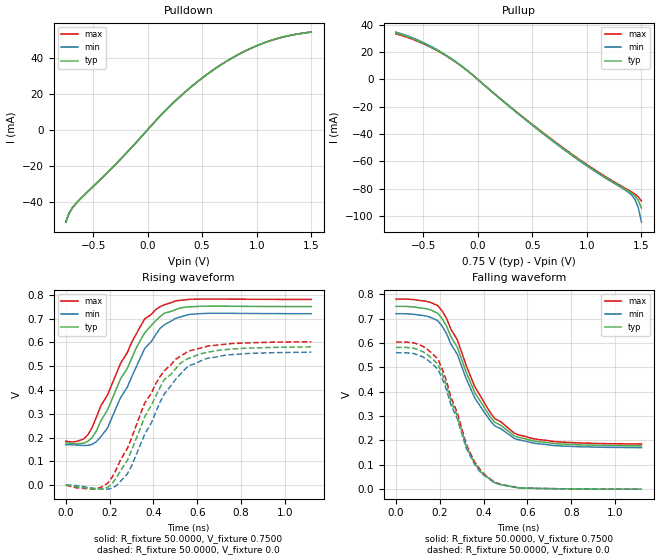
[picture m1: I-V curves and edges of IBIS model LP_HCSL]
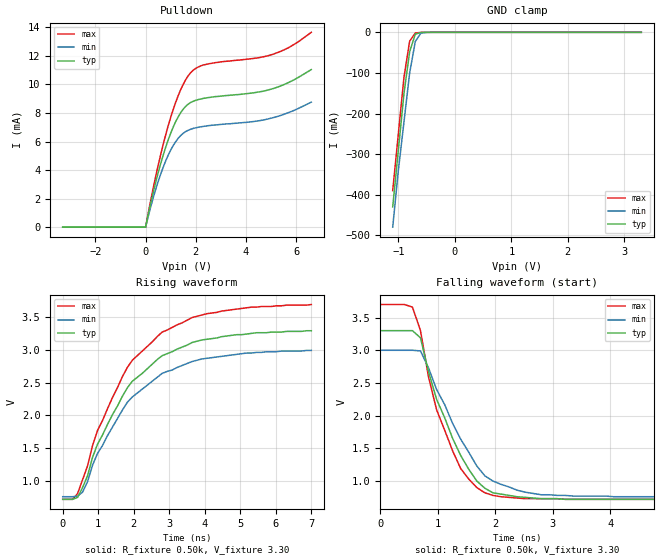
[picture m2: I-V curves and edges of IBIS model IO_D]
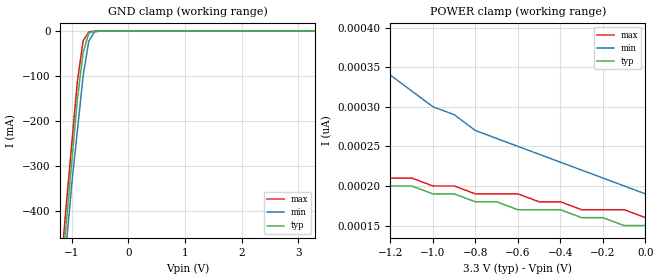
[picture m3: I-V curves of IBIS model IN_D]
| Integrated Devices Technolgy, Inc
[IBIS Ver]   4.1
[File name]   9zxl1530b.ibs
[File Rev]   1.3
|Rev history   1.3   Replace LP_HCSL model
[Date]   June 10, 2015
|[File Rev]   1.0
|Rev history   1.0   original revision
|[Date]   April 4, 2013
[Disclaimer] Integrated Device Technology, Inc. ("IDT") hereby grants the
   user of this ibis model a non-exclusive, nontransferable
   license to use this ibis model under the following terms. the
   user is granted this license only to use the ibis model and is
   not granted rights to sell, copy (except as needed to run the
   ibis model), rent, lease or sub-license the ibis model in
   whole or in part, or in modified form to anyone. the user may
   modify the ibis model to suit its specific applications, but
   rights to derivative works and such modifications shall belong
   to idt. this ibis model is provided on an as is" basis and idt
   makes absolutely no warranty with respect to the information
   contained herein. idt disclaims and customer waives all
   warranties, express and implied, including warranties of
   merchantability and fitness for a particular purpose. the
   entire risk as to quality and performance is with the user
   accordingly, in no event shall idt be liable for any direct or
   indirect damages, whether in contract or tort, including any
   lost profits or other incidental, consequential, exemplary, or
   punitive damages arising out of the use or application of the
   ibis model. further, idt reserves the right to make changes
   without notice to any product herein to improve reliability,
   function, or design. idt does not convey any license under
   patent rights or any other intellectual property rights,
   including those of third parties. idt is not obligated to
   provide maintenance or support for the licensed ibis model.
[Copyright]   Copyright 2012, Integrated Devices Technolgy, Inc. all rights
   reserved
[Notes]
   This file was modified on 6/10/2015 13:07 by the Mentor Graphics
   IBISVTC program, to remove initial non-switching delay(s) from one
   or more models V-t tables. Modified models:
   LP_HCSL,
   IO_D
   Original V-t tables have been left in the affected models, but commented out.
|   COMPONENT: 9ZXL1530B
[Component]   9ZXL1530B
[Manufacturer]   Integrated Device Technology, Inc.
[Package]
| variable   typ   min   max
R_pkg   81.10m   62.20m   100.00m
L_pkg   6.70nH   4.90nH   8.50nH
C_pkg   0.53pF   0.21pF   0.85pF
[Pin]   signal_name   model_name   R_pin   L_pin   C_pin
1   VDDA   POWER
2   GNDA   GND
3   100M_133M#   IN
4   HIBW_BYPM_LOBW#   IN
5   CKPWRGD_PD#   IN
6   GND   GND
7   VDDR   POWER
8   DIF_IN   DIFF_IN
9   DIF_IN#   DIFF_IN
10   SMB_A0_tri   IN
11   SMBDAT   IO_D
12   SMBCLK   IN_D
13   SMB_A1_tri   IN
14   FBOUT_NC#   LP_HCSL
15   FBOUT_NC   LP_HCSL
16   GND   GND
17   DIF_0   LP_HCSL
18   DIF_0#   LP_HCSL
19   VDDIO   POWER
20   GND   GND
21   DIF_1   LP_HCSL
22   DIF_1#   LP_HCSL
23   DIF_2   LP_HCSL
24   DIF_2#   LP_HCSL
25   GND   GND
26   VDD   POWER
27   DIF_3   LP_HCSL
28   DIF_3#   LP_HCSL
29   DIF_4   LP_HCSL
30   DIF_4#   LP_HCSL
31   VDDIO   POWER
32   GND   GND
33   DIF_5   LP_HCSL
34   DIF_5#   LP_HCSL
35   GND   GND
36   VDDIO   POWER
37   DIF_6   LP_HCSL
38   DIF_6#   LP_HCSL
39   DIF_7   LP_HCSL
40   DIF_7#   LP_HCSL
41   VDD   POWER
42   GND   GND
43   DIF_8   LP_HCSL
44   DIF_8#   LP_HCSL
45   DIF_9   LP_HCSL
46   DIF_9#   LP_HCSL
47   GND   GND
48   VDDIO   POWER
49   DIF_10   LP_HCSL
50   DIF_10#   LP_HCSL
51   VDDIO   POWER
52   GND   GND
53   DIF_11   LP_HCSL
54   DIF_11#   LP_HCSL
55   DIF_12   LP_HCSL
56   DIF_12#   LP_HCSL
57   GND   GND
58   VDD   POWER
59   DIF_13   LP_HCSL
60   DIF_13#   LP_HCSL
61   DIF_14   LP_HCSL
62   DIF_14#   LP_HCSL
63   VDDIO   POWER
64   GND   GND
[Diff Pin]   inv_pin   vdiff   tdelay_typ
8   9   NA   NA
15   14   NA   NA
17   18   NA   NA
21   22   NA   NA
23   24   NA   NA
27   28   NA   NA
29   30   NA   NA
33   34   NA   NA
37   38   NA   NA
39   40   NA   NA
43   44   NA   NA
45   46   NA   NA
49   50   NA   NA
53   54   NA   NA
55   56   NA   NA
59   60   NA   NA
61   62   NA   NA
| Models and submodels in the file (5): LP_HCSL (Output), IO_D (I/O_open_drain), IN_D (Input), IN (Input), DIFF_IN (Input)
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|   Model LP_HCSL
[Model]   LP_HCSL
Model_type Output
Polarity   Non-Inverting
Vmeas =  0.4000V
Cref =   2.0000pF
Rref =   0.0
Vref =   0.4000V
C_comp   1.1000pF   1.0000pF   1.2000pF
[Temperature Range]   25.0000   75.0000   0.0000
[Voltage Range]   0.7500V   0.7200V   0.7800V
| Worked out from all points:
|   slope of the pulldown table from 0 to 0.112 V, typ, clamps not added: 15.1 ohm
|   slope of the pullup table from 0 to 0.112 V, typ, clamps not added: 14.4 ohm
|   rising waveform, R_fixture 50.0000, V_fixture 0.7500: 20-80 % time 183ps typ, 186ps min, 189ps max; typ from 0.177 V to 0.75 V
|   rising waveform, R_fixture 50.0000, V_fixture 0.0: 20-80 % time 192ps typ, 189ps min, 192ps max; typ from 0 V to 0.581 V
|   falling waveform, R_fixture 50.0000, V_fixture 0.7500: 20-80 % time 188ps typ, 187ps min, 190ps max; typ from 0.75 V to 0.178 V
|   falling waveform, R_fixture 50.0000, V_fixture 0.0: 20-80 % time 139ps typ, 139ps min, 139ps max; typ from 0.582 V to 0 V
[Pulldown]
|Voltage   I(typ)   I(min)   I(max)
-750mV    -51.3mA    -51.29mA   -51.32mA
-720mV    -46.33mA   -46.32mA   -46.34mA
-690mV    -43.41mA   -43.4mA    -43.42mA
-630mV    -39.24mA   -39.23mA   -39.24mA
-240mV    -15.84mA   -15.84mA   -15.84mA
180mV     11.62mA    11.62mA    11.62mA
330mV     20.18mA    20.18mA    20.18mA
480mV     27.74mA    27.74mA    27.74mA
720mV     37.83mA    37.83mA    37.83mA
990mV     46.31mA    46.31mA    46.31mA
1.23V     51.24mA    51.24mA    51.24mA
1.5V      54.14mA    54.14mA    54.14mA
[Pullup]
|Voltage   I(typ)   I(min)   I(max)
-750mV    34.02mA    34.68mA    33.35mA
-480mV    25.87mA    26.28mA    25.45mA
-240mV    14.89mA    15.08mA    14.69mA
-90mV     6.064mA    6.135mA    5.992mA
360mV     -24.34mA   -24.59mA   -24.09mA
750mV     -48.65mA   -49.09mA   -48.19mA
1.08V     -67.16mA   -67.68mA   -66.63mA
1.38V     -81.8mA    -82.7mA    -81.06mA
1.41V     -83.41mA   -84.74mA   -82.5mA
1.44V     -85.42mA   -87.87mA   -84.07mA
1.47V     -88.51mA   -93.63mA   -86.04mA
1.5V      -94.23mA   -104.6mA   -89.1mA
[Ramp]
| variable   typ   min   max
dV/dt_r  0.3484/0.1898n   0.3352/0.1864n   0.3614/0.1921n
dV/dt_f  0.3432/0.1852n   0.3297/0.1833n   0.3567/0.1870n
R_load = 50.0000
[Rising Waveform]
R_fixture= 50.0000
V_fixture= 0.7500
V_fixture_min= 0.7200
V_fixture_max= 0.7800
|time   V(typ)   V(min)   V(max)
|0.0S   0.1772V   0.1698V   0.1847V
|22.22pS   0.1772V   0.1698V   0.1847V
|44.44pS   0.1772V   0.1698V   0.1847V
|66.67pS   0.1772V   0.1698V   0.1847V
|88.89pS   0.1772V   0.1698V   0.1847V
|0.11nS   0.1772V   0.1698V   0.1847V
|0.13nS   0.1772V   0.1698V   0.1847V
|0.16nS   0.1772V   0.1698V   0.1847V
|0.18nS   0.1772V   0.1698V   0.1847V
|0.20nS   0.1772V   0.1698V   0.1847V
|0.22nS   0.1772V   0.1698V   0.1847V
|0.24nS   0.1772V   0.1698V   0.1847V
|0.27nS   0.1772V   0.1698V   0.1847V
|0.29nS   0.1772V   0.1698V   0.1847V
|0.31nS   0.1772V   0.1698V   0.1847V
|0.33nS   0.1772V   0.1698V   0.1847V
|0.36nS   0.1772V   0.1698V   0.1847V
|0.38nS   0.1772V   0.1698V   0.1847V
|0.40nS   0.1772V   0.1698V   0.1847V
|0.42nS   0.1772V   0.1698V   0.1847V
|0.44nS   0.1772V   0.1698V   0.1847V
|0.47nS   0.1772V   0.1698V   0.1847V
|0.49nS   0.1772V   0.1698V   0.1847V
|0.51nS   0.1772V   0.1698V   0.1847V
|0.53nS   0.1772V   0.1698V   0.1847V
|0.56nS   0.1772V   0.1698V   0.1847V
|0.58nS   0.1772V   0.1698V   0.1847V
|0.60nS   0.1772V   0.1698V   0.1847V
|0.62nS   0.1772V   0.1698V   0.1847V
|0.64nS   0.1772V   0.1698V   0.1847V
|0.67nS   0.1772V   0.1698V   0.1847V
|0.69nS   0.1772V   0.1698V   0.1847V
|0.71nS   0.1772V   0.1698V   0.1847V
|0.73nS   0.1772V   0.1698V   0.1847V
|0.76nS   0.1772V   0.1698V   0.1847V
|0.78nS   0.1772V   0.1698V   0.1847V
|0.80nS   0.1772V   0.1698V   0.1847V
|0.82nS   0.1772V   0.1698V   0.1847V
|0.84nS   0.1772V   0.1698V   0.1847V
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0s        177.2mV    169.8mV    184.7mV
50.33ps   173.6mV    167.9mV    184.1mV
100.3ps   183.7mV    166.7mV    210.9mV
160.3ps   270.8mV    203.9mV    333.6mV
190.3ps   315.9mV    239.9mV    378.7mV
250.3ps   447.1mV    368.1mV    512.4mV
360.3ps   640.1mV    574.6mV    698.3mV
430.3ps   708.2mV    659mV      749.8mV
560.3ps   748.9mV    717mV      780.4mV
1.12ns    750.3mV    720.3mV    780.2mV
[Rising Waveform]
R_fixture= 50.0000
V_fixture= 0.0
V_fixture_min= 0.0
V_fixture_max= 0.0
|time   V(typ)   V(min)   V(max)
|0.0S   0.0V   0.0V   0.0V
|22.22pS   0.0V   0.0V   0.0V
|44.44pS   0.0V   0.0V   0.0V
|66.67pS   0.0V   0.0V   0.0V
|88.89pS   0.0V   0.0V   0.0V
|0.11nS   0.0V   0.0V   0.0V
|0.13nS   0.0V   0.0V   0.0V
|0.16nS   0.0V   0.0V   0.0V
|0.18nS   0.0V   0.0V   0.0V
|0.20nS   0.0V   0.0V   0.0V
|0.22nS   0.0V   0.0V   0.0V
|0.24nS   0.0V   0.0V   0.0V
|0.27nS   0.0V   0.0V   0.0V
|0.29nS   0.0V   0.0V   0.0V
|0.31nS   0.0V   0.0V   0.0V
|0.33nS   0.0V   0.0V   0.0V
|0.36nS   0.0V   0.0V   0.0V
|0.38nS   0.0V   0.0V   0.0V
|0.40nS   0.0V   0.0V   0.0V
|0.42nS   0.0V   0.0V   0.0V
|0.44nS   0.0V   0.0V   0.0V
|0.47nS   0.0V   0.0V   0.0V
|0.49nS   0.0V   0.0V   0.0V
|0.51nS   0.0V   0.0V   0.0V
|0.53nS   0.0V   0.0V   0.0V
|0.56nS   0.0V   0.0V   0.0V
|0.58nS   0.0V   0.0V   0.0V
|0.60nS   0.0V   0.0V   0.0V
|0.62nS   0.0V   0.0V   0.0V
|0.64nS   0.0V   0.0V   0.0V
|0.67nS   0.0V   0.0V   0.0V
|0.69nS   0.0V   0.0V   0.0V
|0.71nS   0.0V   0.0V   0.0V
|0.73nS   0.0V   0.0V   0.0V
|0.76nS   0.0V   0.0V   0.0V
|0.78nS   0.0V   0.0V   0.0V
|0.80nS   0.0V   0.0V   0.0V
|0.82nS   0.0V   0.0V   0.0V
|0.84nS   0.0V   0.0V   0.0V
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0s        0V         0V         0V
140.3ps   -17.07mV   -14.7mV    -16.54mV
230.3ps   28.9mV     -2.684mV   65.71mV
280.3ps   102.2mV    46.14mV    152.8mV
360.3ps   287.3mV    214.6mV    345.6mV
410.3ps   373.7mV    307mV      426.5mV
450.3ps   444.1mV    384mV      481.3mV
560.3ps   532.8mV    501.8mV    563.4mV
740.3ps   570.4mV    547.2mV    593.4mV
1.12ns    580.7mV    558.7mV    602.4mV
[Falling Waveform]
R_fixture= 50.0000
V_fixture= 0.7500
V_fixture_min= 0.7200
V_fixture_max= 0.7800
|time   V(typ)   V(min)   V(max)
|0.0S   0.7500V   0.7200V   0.7800V
|22.22pS   0.7500V   0.7200V   0.7800V
|44.44pS   0.7500V   0.7200V   0.7800V
|66.67pS   0.7500V   0.7200V   0.7800V
|88.89pS   0.7500V   0.7200V   0.7800V
|0.11nS   0.7500V   0.7200V   0.7800V
|0.13nS   0.7500V   0.7200V   0.7800V
|0.16nS   0.7500V   0.7200V   0.7800V
|0.18nS   0.7500V   0.7200V   0.7800V
|0.20nS   0.7500V   0.7200V   0.7800V
|0.22nS   0.7500V   0.7200V   0.7800V
|0.24nS   0.7500V   0.7200V   0.7800V
|0.27nS   0.7500V   0.7200V   0.7800V
|0.29nS   0.7500V   0.7200V   0.7800V
|0.31nS   0.7500V   0.7200V   0.7800V
|0.33nS   0.7500V   0.7200V   0.7800V
|0.36nS   0.7500V   0.7200V   0.7800V
|0.38nS   0.7500V   0.7200V   0.7800V
|0.40nS   0.7500V   0.7200V   0.7800V
|0.42nS   0.7500V   0.7200V   0.7800V
|0.44nS   0.7500V   0.7200V   0.7800V
|0.47nS   0.7500V   0.7200V   0.7800V
|0.49nS   0.7500V   0.7200V   0.7800V
|0.51nS   0.7500V   0.7200V   0.7800V
|0.53nS   0.7500V   0.7200V   0.7800V
|0.56nS   0.7500V   0.7200V   0.7800V
|0.58nS   0.7500V   0.7200V   0.7800V
|0.60nS   0.7500V   0.7200V   0.7800V
|0.62nS   0.7500V   0.7200V   0.7800V
|0.64nS   0.7500V   0.7200V   0.7800V
|0.67nS   0.7500V   0.7200V   0.7800V
|0.69nS   0.7500V   0.7200V   0.7800V
|0.71nS   0.7500V   0.7200V   0.7800V
|0.73nS   0.7500V   0.7200V   0.7800V
|0.76nS   0.7500V   0.7200V   0.7800V
|0.78nS   0.7500V   0.7200V   0.7800V
|0.80nS   0.7500V   0.7200V   0.7800V
|0.82nS   0.7500V   0.7200V   0.7800V
|0.84nS   0.7500V   0.7200V   0.7800V
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0s        750mV      720mV      780mV
140.3ps   740.3mV    710.1mV    770.6mV
190.3ps   722.3mV    691.6mV    753.3mV
230.3ps   669.8mV    638.9mV    701.7mV
280.3ps   581.5mV    552.3mV    612.1mV
360.3ps   395.2mV    372.9mV    419mV
450.3ps   275mV      260.4mV    290.2mV
540.3ps   218.6mV    208.1mV    229.8mV
720.3ps   187.6mV    179.2mV    195.7mV
1.12ns    178mV      170.5mV    185.5mV
[Falling Waveform]
R_fixture= 50.0000
V_fixture= 0.0
V_fixture_min= 0.0
V_fixture_max= 0.0
|time   V(typ)   V(min)   V(max)
|0.0S   0.5818V   0.5599V   0.6034V
|22.22pS   0.5818V   0.5599V   0.6034V
|44.44pS   0.5818V   0.5599V   0.6034V
|66.67pS   0.5818V   0.5599V   0.6034V
|88.89pS   0.5818V   0.5599V   0.6034V
|0.11nS   0.5818V   0.5599V   0.6034V
|0.13nS   0.5818V   0.5599V   0.6034V
|0.16nS   0.5818V   0.5599V   0.6034V
|0.18nS   0.5818V   0.5599V   0.6034V
|0.20nS   0.5818V   0.5599V   0.6034V
|0.22nS   0.5818V   0.5599V   0.6034V
|0.24nS   0.5818V   0.5599V   0.6034V
|0.27nS   0.5818V   0.5599V   0.6034V
|0.29nS   0.5818V   0.5599V   0.6034V
|0.31nS   0.5818V   0.5599V   0.6034V
|0.33nS   0.5818V   0.5599V   0.6034V
|0.36nS   0.5818V   0.5599V   0.6034V
|0.38nS   0.5818V   0.5599V   0.6034V
|0.40nS   0.5818V   0.5599V   0.6034V
|0.42nS   0.5818V   0.5599V   0.6034V
|0.44nS   0.5818V   0.5599V   0.6034V
|0.47nS   0.5818V   0.5599V   0.6034V
|0.49nS   0.5818V   0.5599V   0.6034V
|0.51nS   0.5818V   0.5599V   0.6034V
|0.53nS   0.5818V   0.5599V   0.6034V
|0.56nS   0.5818V   0.5599V   0.6034V
|0.58nS   0.5818V   0.5599V   0.6034V
|0.60nS   0.5818V   0.5599V   0.6034V
|0.62nS   0.5818V   0.5599V   0.6034V
|0.64nS   0.5818V   0.5599V   0.6034V
|0.67nS   0.5818V   0.5599V   0.6034V
|0.69nS   0.5818V   0.5599V   0.6034V
|0.71nS   0.5818V   0.5599V   0.6034V
|0.73nS   0.5818V   0.5599V   0.6034V
|0.76nS   0.5818V   0.5599V   0.6034V
|0.78nS   0.5818V   0.5599V   0.6034V
|0.80nS   0.5818V   0.5599V   0.6034V
|0.82nS   0.5818V   0.5599V   0.6034V
|0.84nS   0.5818V   0.5599V   0.6034V
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0s        581.8mV    559.9mV    603.4mV
100.3ps   572.8mV    550.9mV    594.8mV
190.3ps   514.1mV    493.6mV    535.2mV
230.3ps   425.8mV    408.1mV    444.7mV
320.3ps   177.3mV    169mV      186.9mV
340.3ps   139.9mV    133.9mV    146.7mV
390.3ps   68.23mV    64.37mV    73.06mV
450.3ps   26.95mV    25.58mV    28.61mV
560.3ps   5.626mV    5.468mV    5.856mV
1.12ns    174.6uV    171.5uV    178.3uV
|   Model IO_D
[Model]   IO_D
Model_type   I/O_open_drain
Polarity   Inverting
Enable   Active-High
Vinl =   0.80V
Vinh =   2.00V
Vmeas =   1.50V
Cref =   5.00pF
Rref =  0.000
Vref =   1.50V
C_comp   3.40pF   2.85pF   3.95pF
[Temperature Range]   27.00   70.00   0.000
[Voltage Range]   3.30V   3.00V   3.70V
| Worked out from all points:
|   slope of the pulldown table from 0 to 0.495 V, typ, clamps not added: 131 ohm
|   GND clamp passes 1 mA (typ) near -0.62 V on its own axis
|   rising waveform, R_fixture 0.50k, V_fixture 3.30: 20-80 % time 1.74ns typ, 1.76ns min, 1.73ns max; typ from 0.72 V to 3.29 V
|   falling waveform, R_fixture 0.50k, V_fixture 3.30: 20-80 % time 693ps typ, 785ps min, 596ps max; typ from 3.3 V to 0.72 V
[Pulldown]
| voltage   I(typ)   I(min)   I(max)
-3.3V     0A         0A         0A
0V        0A         0A         0A
500mV     3.8mA      3.19mA     4.32mA
900mV     6.11mA     5.04mA     7.1mA
1.2V      7.4mA      5.99mA     8.75mA
1.4V      8.03mA     6.42mA     9.64mA
1.8V      8.74mA     6.86mA     10.83mA
2.1V      8.94mA     7mA        11.22mA
2.5V      9.08mA     7.11mA     11.44mA
5.1V      9.72mA     7.68mA     12.13mA
5.7V      10.14mA    8.03mA     12.58mA
6.6V      11.04mA    8.76mA     13.65mA
[GND_clamp]
| voltage   I(typ)   I(min)   I(max)
  |-3.30   -3.78A   -3.64A   -3.87A
  |-3.20   -3.62A   -3.50A   -3.71A
  |-3.10   -3.47A   -3.35A   -3.55A
  |-3.00   -3.31A   -3.21A   -3.39A
  |-2.90   -3.16A   -3.06A   -3.23A
  |-2.80   -3.01A   -2.91A   -3.07A
  |-2.70   -2.85A   -2.77A   -2.91A
  |-2.60   -2.70A   -2.62A   -2.75A
  |-2.50   -2.54A   -2.48A   -2.59A
  |-2.40   -2.39A   -2.33A   -2.43A
  |-2.30   -2.24A   -2.19A   -2.27A
  |-2.20   -2.08A   -2.04A   -2.11A
  |-2.10   -1.93A   -1.90A   -1.95A
  |-2.00   -1.78A   -1.75A   -1.79A
  |-1.90   -1.62A   -1.61A   -1.63A
  |-1.80   -1.47A   -1.46A   -1.47A
  |-1.70   -1.32A   -1.32A   -1.32A
  |-1.60   -1.17A   -1.18A   -1.16A
  |-1.50   -1.02A   -1.03A   -1.00A
  |-1.40   -0.87A   -0.89A   -0.85A
  |-1.30   -0.72A   -0.75A   -0.69A
  |-1.20   -0.57A   -0.61A   -0.54A
-1.1V     -430mA     -480mA     -390mA
-1V       -290mA     -340mA     -250mA
-900mV    -150mA     -220mA     -110mA
-800mV    -47.73mA   -100mA     -21.74mA
-700mV    -4.4mA     -22.46mA   -1.7mA
-600mV    -390uA     -1.82mA    -190uA
-400mV    -1.59uA    -9.25uA    -420nA
3.3V      150pA      220pA      150pA
[Ramp]
| variable   typ   min   max
dV/dt_r   0.27/0.19n   0.21/0.19n   0.35/0.18n
dV/dt_f   0.27/0.21n   0.21/0.22n   0.35/0.20n
[Rising Waveform]
R_fixture = 0.50k
V_fixture = 3.30
V_fixture_min = 3.00
V_fixture_max = 3.70
| time   V(typ)   V(min)   V(max)
0s        720mV      760mV      720mV
280ps     720mV      760mV      720mV
420ps     750mV      770mV      810mV
560ps     900mV      830mV      1.02V
700ps     1.08V      990mV      1.23V
980ps     1.56V      1.42V      1.77V
1.82ns    2.42V      2.2V       2.73V
2.8ns     2.91V      2.64V      3.27V
4.06ns    3.16V      2.87V      3.55V
7ns       3.29V      2.99V      3.69V
[Falling Waveform]
R_fixture = 0.50k
V_fixture = 3.30
V_fixture_min = 3.00
V_fixture_max = 3.70
| time   V(typ)   V(min)   V(max)
0s        3.3V       3V         3.7V
560ps     3.3V       3V         3.66V
700ps     3.19V      2.99V      3.3V
840ps     2.67V      2.73V      2.59V
980ps     2.25V      2.4V       2.09V
1.4ns     1.39V      1.64V      1.19V
1.68ns    1V         1.23V      900mV
1.82ns    890mV      1.08V      820mV
2.8ns     730mV      790mV      730mV
7ns       720mV      760mV      720mV
|   Model IN_D
[Model]   IN_D
Model_type   Input
Polarity   Inverting
Enable   Active-High
Vinl =   1.00V
Vinh =   2.00V
C_comp   3.40pF   2.85pF   3.95pF
[Temperature Range]   27.00   70.00   0.000
[Voltage Range]   3.30V   3.00V   3.60V
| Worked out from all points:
|   GND clamp passes 1 mA (typ) near -0.62 V on its own axis
[GND_clamp]
| voltage   I(typ)   I(min)   I(max)
-3.3V     -3.78A     -3.65A     -3.87A
-1.2V     -570mA     -610mA     -540mA
-1.1V     -430mA     -480mA     -390mA
-1V       -290mA     -340mA     -250mA
-900mV    -150mA     -220mA     -110mA
-800mV    -47.77mA   -100mA     -21.77mA
-700mV    -4.42mA    -22.5mA    -1.71mA
-600mV    -390uA     -1.83mA    -190uA
-500mV    -33.14uA   -140uA     -13.41uA
3.3V      150pA      220pA      150pA
[POWER_clamp]
| voltage   I(typ)   I(min)   I(max)
-3.3V     350pA      1.67nA     300pA
-2.6V     280pA      890pA      270pA
-2.5V     280pA      820pA      260pA
-2.3V     260pA      700pA      260pA
-2.2V     250pA      640pA      250pA
-1.5V     220pA      400pA      220pA
-1.4V     210pA      380pA      220pA
-1V       190pA      300pA      200pA
-800mV    180pA      270pA      190pA
-600mV    170pA      250pA      190pA
-400mV    170pA      230pA      180pA
0V        150pA      190pA      160pA
